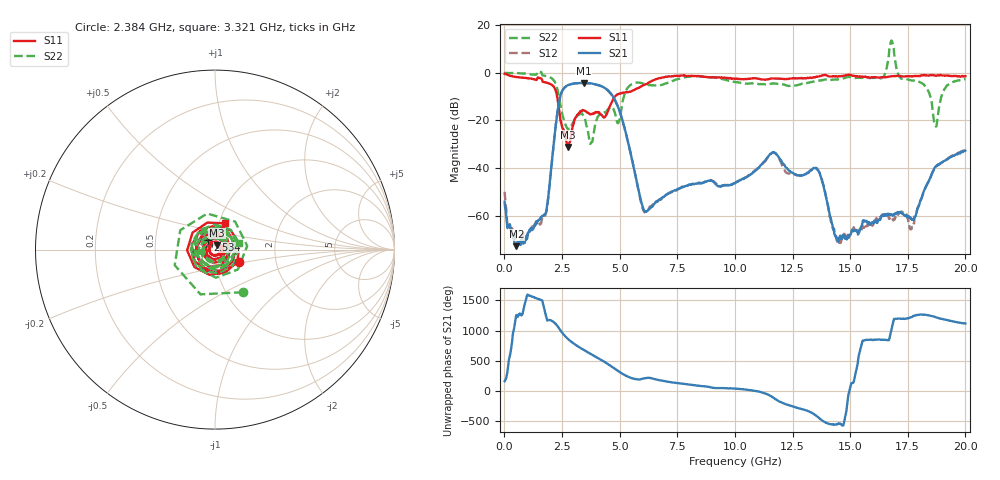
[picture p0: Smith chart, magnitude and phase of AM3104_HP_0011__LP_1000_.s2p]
!Created with skrf (http://scikit-rf.org).
# Hz S RI R 50.0
!freq ReS11 ImS11 ReS21 ImS21 ReS12 ImS12 ReS22 ImS22
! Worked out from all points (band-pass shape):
!   1601 points, 10 MHz to 20 GHz, reference 50 ohm
!   highest |S21| = -4.24 dB at 3.433 GHz (marker M1); lowest = -72.8 dB at 522.2 MHz (marker M2)
!   |S21| within 3 dB of the highest: 2.528 GHz to 4.485 GHz (1.957 GHz wide, 55.8 % of centre)
!   lowest |S11| = -31.1 dB at 2.759 GHz (marker M3), VSWR 1.06, Z = 51.1 + j2.61 ohm
!   |S11| at or under -10 dB: 2.29 GHz to 4.789 GHz (2.499 GHz wide, 70.6 % of centre)
!   |S22| runs from -29.9 to 13.6 dB; largest |S21 - S12| = 0.044
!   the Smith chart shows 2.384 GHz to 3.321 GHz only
!   S11 on the Smith chart (normalised r, x): 2.384 GHz: 1.30, -0.18; 2.534 GHz: 0.92, +0.10; 3.321 GHz: 1.07, +0.32
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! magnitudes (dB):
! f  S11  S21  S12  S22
! 10 MHz  -0.4  -54.2  -50.0  0.0
! 522.2 MHz  -1.7  -72.8  -70.5  -0.1
! 1.784 GHz  -4.0  -59.1  -59.4  -1.2
! 2.384 GHz  -16.4  -11.6  -11.7  -10.9
! 2.534 GHz  -23.5  -7.1  -7.2  -18.2
! 2.759 GHz  -31.1  -5.2  -5.2  -23.8
! 3.321 GHz  -16.1  -4.3  -4.4  -17.0
! 3.346 GHz  -15.9  -4.3  -4.4  -16.9
! 3.433 GHz  -15.8  -4.2  -4.3  -18.4
! 3.758 GHz  -17.3  -4.4  -4.5  -29.2
! 4.708 GHz  -11.3  -9.8  -10.0  -14.8
! 6.007 GHz  -5.3  -56.5  -57.4  -4.5
! 6.682 GHz  -2.3  -53.5  -53.7  -5.3
! 10.01 GHz  -2.5  -46.4  -46.3  -3.9
! 11.64 GHz  -2.4  -33.5  -33.5  -4.4
! 13.34 GHz  -2.1  -40.6  -40.7  -3.8
! 14.5 GHz  -1.4  -70.8  -71.4  -2.8
! 16.68 GHz  -1.6  -59.4  -61.1  7.2
! 17.68 GHz  -1.5  -61.8  -65.3  -3.2
! 18.7 GHz  -1.2  -39.4  -39.6  -22.2
! 19.14 GHz  -1.1  -36.8  -36.6  -6.3
! 20 GHz  -1.4  -32.7  -32.2  -2.6
